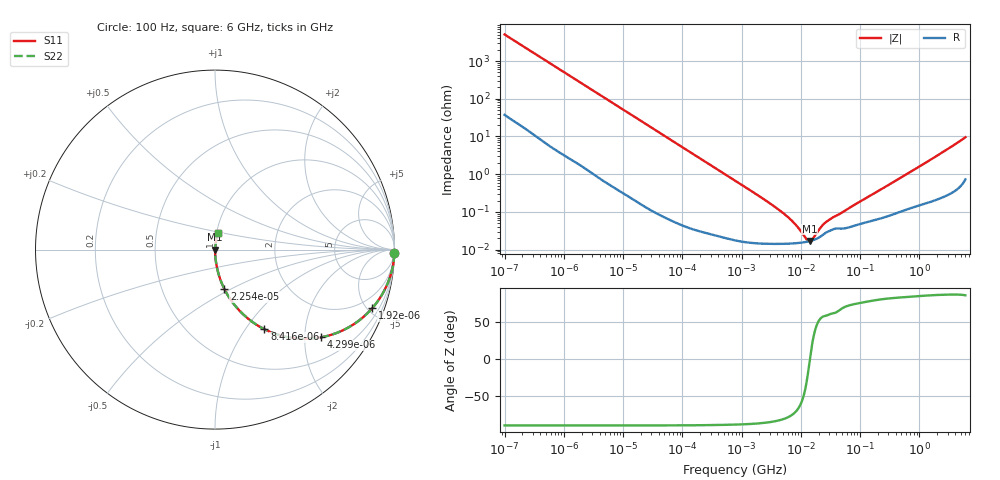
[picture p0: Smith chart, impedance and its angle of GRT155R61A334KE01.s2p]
!Murata Part Number: GRT155R61A334KE01
!These Parameters are Measured in Series Mode Connection
!Data Generated on Jun 19, 2026
!  o--ll--o
!Port1  Port2
!  o------o
!Operation Temp=25[degC], DC Bias Voltage=0[V]
!Freq. Start=100[Hz] Stop=6[GHz] 401[Steps]
# Hz S RI R 50
!Freq.(Hz) S11(Real) S11(Imag) S21(Real) S21(Imag) S12(Real) S12(Imag) S22(Real) S22(Imag)
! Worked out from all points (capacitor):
!   401 points, 100 Hz to 6 GHz, reference 50 ohm
!   read as one part in series: C = 313 nF near 109 Hz
!   lowest |Z| = 16.8 mohm at 14.22 MHz (marker M1)
!   series resonance near 14.27 MHz, so ESL is about 400 pH
!   S11 on the Smith chart (normalised r, x): 100 Hz: open; 1.92 kHz: 1.03, -5.35; 4.299 kHz: 1.01, -2.40; 8.416 kHz: 1.01, -1.23; 22.54 kHz: 1.00, -0.46; 6 GHz: 1.01, +0.19
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100  0.9995 -0.0197  0.000533 0.0197  0.000533 0.0197  0.9995 -0.0197
548  0.988 -0.1058  0.012 0.1058  0.012 0.1058  0.988 -0.1058
1122  0.9531 -0.2083  0.0469 0.2083  0.0469 0.2083  0.9531 -0.2083
1920  0.8759 -0.3266  0.1241 0.3266  0.1241 0.3266  0.8759 -0.3266
2008  0.866 -0.3375  0.134 0.3375  0.134 0.3375  0.866 -0.3375
4299  0.5892 -0.489  0.4108 0.489  0.4108 0.489  0.5892 -0.489
8416  0.275 -0.4435  0.725 0.4435  0.725 0.4435  0.275 -0.4435
13169  0.1353 -0.339  0.8647 0.339  0.8647 0.339  0.1353 -0.339
22537  0.0515 -0.218  0.9485 0.218  0.9485 0.218  0.0515 -0.218
40335  0.0171 -0.1265  0.9829 0.1265  0.9829 0.1265  0.0171 -0.1265
129199  0.002 -0.0403  0.998 0.0403  0.998 0.0403  0.002 -0.0403
774597  0.000221 -0.00677  0.9998 0.00677  0.9998 0.00677  0.000221 -0.00677
5079039  0.000143 -0.000907  0.9999 0.000907  0.9999 0.000907  0.000143 -0.000907
7947587  0.000147 -0.000458  0.9999 0.000458  0.9999 0.000458  0.000147 -0.000458
1.243624e7  0.00016 -0.000102  0.9998 0.000102  0.9998 0.000102  0.00016 -0.000102
1.422411e7  0.000168 -2.4e-06  0.9998 2.4e-06  0.9998 2.4e-06  0.000168 -2.4e-06
1.555665e7  0.000175 6.4e-05  0.9998 -6.4e-05  0.9998 -6.4e-05  0.000175 6.4e-05
2.225763e7  0.00023 0.000335  0.9998 -0.000335  0.9998 -0.000335  0.00023 0.000335
2.911731e7  0.000302 0.000509  0.9997 -0.000509  0.9997 -0.000509  0.000302 0.000509
3.124326e8  0.000819 0.00527  0.9992 -0.00527  0.9992 -0.00527  0.000819 0.00527
1.873145e9  0.00287 0.0289  0.9971 -0.0289  0.9971 -0.0289  0.00287 0.0289
6e9  0.016 0.0928  0.984 -0.0928  0.984 -0.0928  0.016 0.0928
